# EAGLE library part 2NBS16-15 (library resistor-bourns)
BOURNS RESISTOR NETWORK
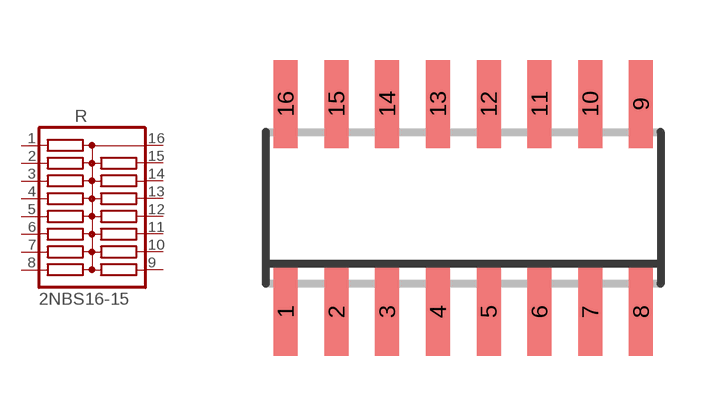
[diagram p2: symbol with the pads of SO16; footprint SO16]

Designator prefix R

## 2NBS16-15 (OC_FARNELL: unknown; OC_NEWARK: unknown)  [SO16]
1  1  pas
2  2  pas
3  3  pas
4  4  pas
5  5  pas
6  6  pas
7  7  pas
8  8  pas
9  9  pas
10  10  pas
11  11  pas
12  12  pas
13  13  pas
14  14  pas
15  15  pas
16  16  pas

## Footprint SO16 (pad centres in mm)
BOURNS RESISTOR NETWORK
smd 0.6 x 2.2: 1 -4.445,-2.6; 2 -3.175,-2.6; 3 -1.905,-2.6; 4 -0.635,-2.6; 5 0.635,-2.6; 6 1.905,-2.6; 7 3.175,-2.6; 8 4.445,-2.6; 9 4.445,2.6; 10 3.175,2.6; 11 1.905,2.6; 12 0.635,2.6; 13 -0.635,2.6; 14 -1.905,2.6; 15 -3.175,2.6; 16 -4.445,2.6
